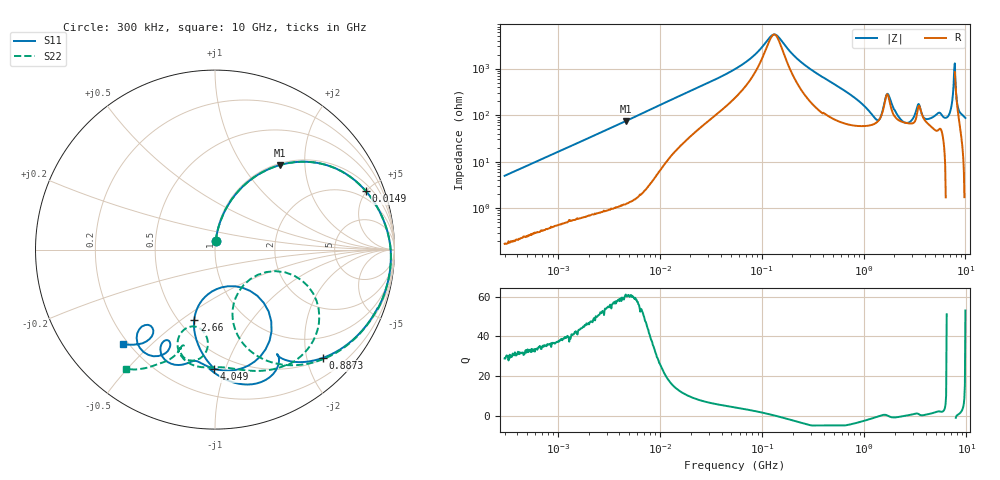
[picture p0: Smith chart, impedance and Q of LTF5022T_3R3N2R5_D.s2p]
! S-Parameter Data Generated by TDK Corporation
! Copyright(C) 2020 TDK Corporation.
! All Rights Reserved.
! TDK P/N: LTF5022T-3R3N2R5-D (Inductor)
! Property: L=3.3uH at 100kHz
! Size(LxWxT): 6.5x5x2.2mm
! Model Type: s2p (Touchstone File Format Version 1.0)
! Frequency: DC=Yes Start=0.3MHz Stop=10000MHz 802points Log-sweep
! Model Generated on Apr. 23, 2020
! Port Assignments:
!  1 ---@@@--- 2
! Applicable Conditions:
!  Temperature = 25 degC
!  DC Bias Current = 0 A
!  Small Signal Operation
! Terms and conditions regarding TDK Simulation Models
! (1)This simulation model is being provided solely for informational purposes. Please refer to the specifications of the products in terms of detailed characteristics of such products.
! (2)In no event shall TDK Corporation of any of its subsidiaries be liable for any loss or damage arising, directly or indirectly,
!  From any information contained in this simulation model, including, but not limited to loss or damages arising from any inaccuracies, omissions or errors in connection with such information.
! (3)Any and all copyrights on this simulation model are owned by TDK Corporation.
!  Duplication or redistribution of this simulation model without prior written permission from TDK Corporation is prohibited.
! (4)This simulation model is subject to any modification or change without any prior notice.
! (5)Neither TDK Corporation nor any of its subsidiaries shall make any warranty, express or implied,
!  Including but not limited to the correctness, implied warranties of merchantability and fitness for a particular purpose with respect to this simulation models.
! (6)The use of this simulation model shall be deemed to have consented to the terms and conditions hereof.
# Hz S MA R 50
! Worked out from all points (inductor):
!   801 points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, 300 kHz to 10 GHz, reference 50 ohm
!   read as one part in series: L = 2.63 uH near 318.3 kHz
!   highest Q = 60.4 at 4.673 MHz (marker M1), where L = 2.56 uH
!   self-resonance near 132.6 MHz
!   S11 on the Smith chart (normalised r, x): 300 kHz: 1.00, +0.10; 14.9 MHz: 1.43, +4.98; 887.3 MHz: 0.53, -2.32; 2.66 GHz: 0.60, -0.56; 4.049 GHz: 0.39, -0.91; 10 GHz: 0.18, -0.41
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300000  0.04977 85.3  0.997 -2.8  0.997 -2.8  0.04979 85.1
1713600  0.2644 73.3  0.9584 -15.4  0.9584 -15.4  0.2643 73.3
4673027  0.5951 52.4  0.7938 -36.7  0.7938 -36.6  0.5951 52.4
9671944  0.8321 31.4  0.5253 -56.5  0.5253 -56.6  0.8321 31.4
1.49005e7  0.9023 21.1  0.3676 -64.6  0.3676 -64.6  0.9023 21.0
5.477226e7  0.9712 4.0  0.09974 -72.2  0.09976 -72.2  0.9712 3.9
1.340254e8  0.9816 -4.0  0.01816 -0.6  0.01816 -0.7  0.9817 -4.2
3.126428e8  0.9746 -14.9  0.1044 63.8  0.1043 63.8  0.9742 -15.6
8.872678e8  0.8525 -45.0  0.3496 28.3  0.3495 28.3  0.8314 -49.2
1.371335e9  0.6782 -59.4  0.4755 -21.0  0.4764 -20.9  0.3985 -75.6
1.569319e9  0.743 -62.1  0.3334 -49.2  0.3355 -49.3  0.3583 -19.6
1.767019e9  0.7669 -78.2  0.2068 -20.9  0.2062 -21.6  0.7092 -35.3
2.020878e9  0.6634 -90.4  0.3358 -17.1  0.3338 -17.3  0.7553 -58.4
2.659614e9  0.4074 -106.5  0.4165 -54.2  0.4138 -54.3  0.6661 -82.7
3.135132e9  0.2134 -79.4  0.3414 -83.8  0.3377 -83.6  0.6584 -95.1
3.472057e9  0.5074 -51.9  0.1948 -76.2  0.1947 -75.0  0.6045 -109.4
4.049484e9  0.6638 -90.5  0.3609 -79.6  0.3615 -79.6  0.4439 -105.3
5.040844e9  0.6527 -103.8  0.3241 -127.8  0.3219 -127.7  0.5427 -94.3
6.737565e9  0.5773 -115.7  0.2355 -179.5  0.2334 -178.1  0.5689 -107.9
7.875699e9  0.6896 -127.4  0.0151 -30.6  0.008036 -66.1  0.6155 -110.1
8.770142e9  0.5559 -130.1  0.1593 -133.5  0.1526 -134.9  0.7035 -115.7
1e10  0.733 -134.4  0.169 163.5  0.1645 164.4  0.8277 -126.6
